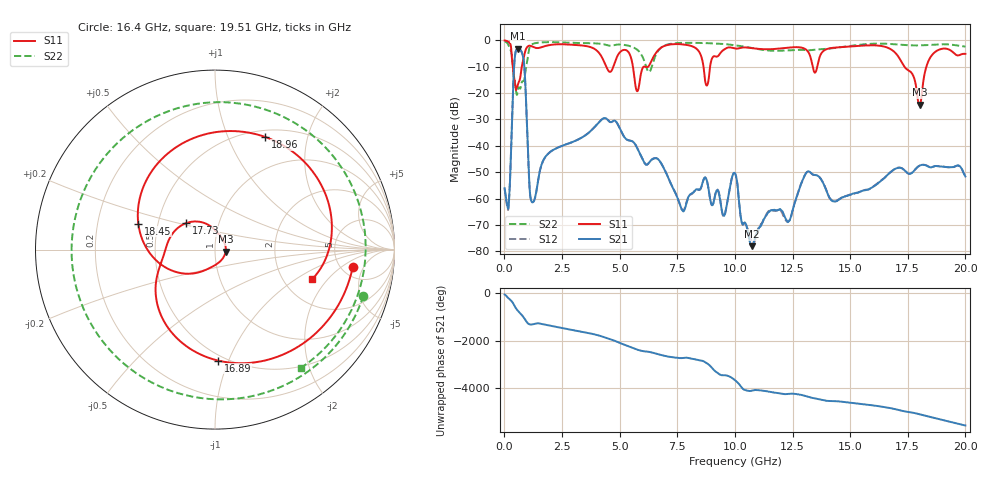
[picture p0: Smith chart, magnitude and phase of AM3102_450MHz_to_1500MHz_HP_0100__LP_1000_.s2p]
!Agilent Technologies,E8364B,MY43040894,A.07.50.67
!Agilent E8364B: A.07.50.67
!Date: Thursday, January 11, 2018 05:37:12
!Correction: S11(Full 2 Port(1,2))
!S21(Full 2 Port(1,2))
!S12(Full 2 Port(1,2))
!S22(Full 2 Port(1,2))
!S2P File: Measurements: S11, S21, S12, S22:
# Hz S  dB  R 50
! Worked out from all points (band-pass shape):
!   1601 points, 10 MHz to 20 GHz, reference 50 ohm
!   highest |S21| = -3.22 dB at 597.2 MHz (marker M1); lowest = -78.0 dB at 10.74 GHz (marker M2)
!   |S21| within 3 dB of the highest: 456.1 MHz to 807.7 MHz (351.6 MHz wide, 55.6 % of centre)
!   lowest |S11| = -24.4 dB at 18.01 GHz (marker M3), VSWR 1.13, Z = 56.3 - j1.27 ohm
!   |S11| at or under -10 dB: 365.3 MHz to 755.9 MHz (390.7 MHz wide, 69.7 % of centre); 5.577 GHz to 6.045 GHz (468.1 MHz wide, 8.05 % of centre); 17.36 GHz to 18.31 GHz (951.1 MHz wide, 5.33 % of centre)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
!   |S22| runs from -20.7 to -0.4 dB; largest |S21 - S12| = 0.002
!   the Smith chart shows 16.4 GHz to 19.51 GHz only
!   S11 on the Smith chart (normalised r, x): 16.4 GHz: 6.31, -3.07; 16.89 GHz: 0.46, -0.92; 17.73 GHz: 0.70, +0.21; 18.45 GHz: 0.39, +0.14; 18.96 GHz: 0.58, +1.38; 19.51 GHz: 2.87, -1.39
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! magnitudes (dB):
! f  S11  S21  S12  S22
! 10 MHz  -0.1  -56.1  -56.2  -0.4
! 184.9 MHz  -0.6  -62.9  -62.4  -2.0
! 434.8 MHz  -14.8  -8.3  -8.3  -14.6
! 597.2 MHz  -16.4  -3.2  -3.2  -18.1
! 834.6 MHz  -6.8  -7.5  -7.5  -15.4
! 1.209 GHz  -2.4  -61.4  -61.2  -1.5
! 3.346 GHz  -2.0  -36.9  -36.9  -1.1
! 5.77 GHz  -19.3  -41.0  -40.9  -3.6
! 6.682 GHz  -3.7  -45.2  -45.2  -3.8
! 7.744 GHz  -1.6  -64.7  -64.6  -1.0
! 10.01 GHz  -3.1  -50.4  -50.5  -1.9
! 10.74 GHz  -3.0  -78.0  -76.7  -2.9
! 13.34 GHz  -8.6  -50.6  -50.7  -3.7
! 16.4 GHz  -2.2  -52.8  -52.8  -1.3
! 16.68 GHz  -3.0  -50.5  -50.6  -1.3
! 16.89 GHz  -4.2  -49.0  -49.0  -1.5
! 17.73 GHz  -13.2  -49.9  -49.8  -1.9
! 18.01 GHz  -24.4  -47.5  -47.5  -1.9
! 18.45 GHz  -6.9  -48.1  -48.1  -1.7
! 18.96 GHz  -3.3  -47.9  -47.8  -1.5
! 19.51 GHz  -4.9  -47.9  -48.0  -1.8
! 20 GHz  -5.1  -51.6  -51.3  -2.4
